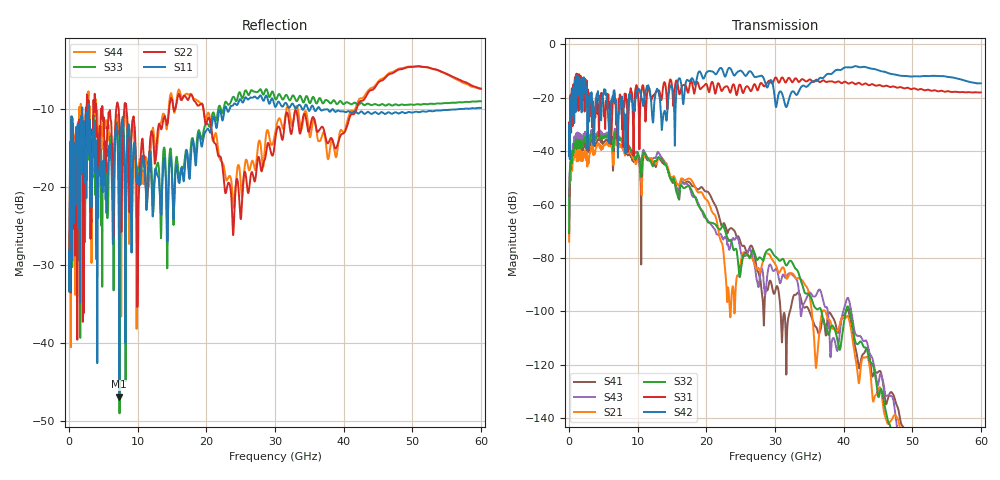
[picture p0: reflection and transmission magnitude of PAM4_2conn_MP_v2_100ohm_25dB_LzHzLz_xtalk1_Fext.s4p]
! Info: Touchstone file created by Circ.  Input file=FAB50GbE_2conn_Midplane_Examax_Topo2_v2_100ohm_25dB_LzHzLz.circ
# Hz S RI R 50
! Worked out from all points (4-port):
!   6000 points, 10 MHz to 60 GHz, reference 50 ohm
!   strongest paths, dB at 10 MHz, 15.01 GHz, 30.01 GHz, 45.01 GHz, 60 GHz:
!     S42: -41.8, -15.8, -21.2, -9.7, -14.6
!     S31: -41.4, -16.1, -12.6, -15.3, -18.0
!     S32: -70.5, -51.0, -79.4, -131.5, -169.4
!     S21: -73.9, -49.6, -82.2, -129.3, -165.3
!     S43: -71.6, -50.8, -84.4, -127.7, -168.9
!     S41: -69.4, -51.4, -92.7, -122.8, -167.3
!   lowest |S11| = -46.8 dB at 7.31 GHz (marker M1), VSWR 1.01, Z = 50.5 + j0.023 ohm
!   |S11| at or under -10 dB: start of sweep to 1.899 GHz; 2.844 GHz to 22.67 GHz (19.83 GHz wide, 155 % of centre); 36.57 GHz to 57.4 GHz (20.83 GHz wide, 44.3 % of centre)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
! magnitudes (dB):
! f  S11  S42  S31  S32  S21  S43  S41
! 10 MHz  -31.1  -41.8  -41.4  -70.5  -73.9  -71.6  -69.4
! 1.01 GHz  -12.6  -14.6  -14.2  -35.7  -38.2  -33.4  -35.0
! 7.31 GHz  -46.8  -25.9  -21.5  -35.7  -38.2  -34.6  -37.3
! 10.07 GHz  -19.4  -16.5  -19.8  -41.0  -41.9  -41.4  -42.5
! 17.74 GHz  -16.4  -13.1  -13.8  -54.1  -50.6  -55.1  -52.3
! 24.83 GHz  -8.8  -10.0  -15.1  -87.0  -84.7  -75.0  -72.9
! 60 GHz  -9.9  -14.6  -18.0  -169.4  -165.3  -168.9  -167.3
